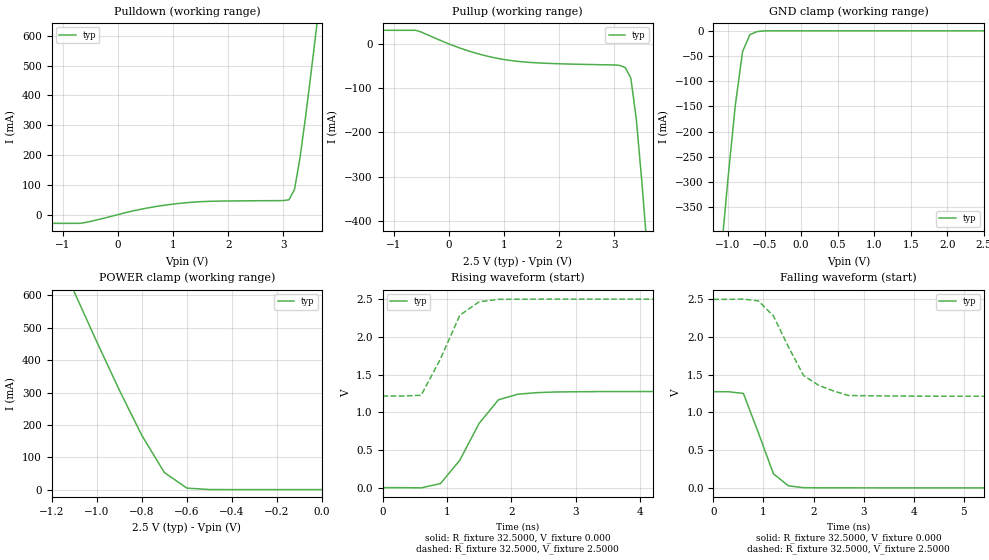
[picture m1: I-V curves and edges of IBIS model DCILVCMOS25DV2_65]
| / 7\'7
| \ \   Xilinx Inc.
| / /
| \_\/.\   IBIS Model for Virtex-II
[IBIS ver]   2.1
[File name]   dci2565d.ibs
[File Rev]   1.1
[Date]   Aug. 1, 2001
[Source]   Hspice simulations (08-01: TT, SS, FF)
[Notes]   Xilinx IBIS model for LVDCI 2.5V 32.5 ohms (65/2) driver
[Disclaimer] The data in this model is derived from SPICE simulations using
   modeling information extracted from the target process. While
   a great deal of care has been taken to provide information
   that is accurate, this model is considered preliminary as it
   has not been verified by actual silicon measurement. Treat the
   data in this model as preliminary until actual silicon
   verification is performed.
[Copyright]   Copyright 2001, Xilinx Inc., All rights reserved
|   Component Virtex_II
[Component]   Virtex_II
[Manufacturer]   Xilinx Inc.
[Package]
| variable   typ   min   max
R_pkg   0.1000   NA   NA
L_pkg   0.8000nH   NA   NA
C_pkg   0.5000pF   NA   NA
[Pin]  signal_name   model_name   R_pin   L_pin   C_pin
io   DCILVCMOS25DV2_65   DCILVCMOS25DV2_65
| ins  insig   inp
| ens  ensig   inp
PGND   GND   GND
VCCO   VCCO   POWER
| Models and submodels in the file (1): DCILVCMOS25DV2_65 (I/O)
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|   Model DCILVCMOS25DV2_65
[Model]   DCILVCMOS25DV2_65
Model_type   I/O
Polarity   Non-Inverting
Enable   Active-Low
Vinh = 1.7V
Vinl = 0.7V
Vmeas =   1.2000V
Cref =  35.0000pF
Rref =   1.0000M
Vref =  0.000V
C_comp   7.0000pF   NA   NA
[Temperature Range]   25.0000   NA   NA
[Voltage Range]   2.5000V   NA   NA
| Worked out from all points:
|   slope of the pulldown table from 0 to 0.375 V, typ, clamps not added: 22.9 ohm
|   slope of the pullup table from 0 to 0.375 V, typ, clamps not added: 22.5 ohm
|   GND clamp passes 1 mA (typ) near -0.57 V on its own axis
|   POWER clamp passes 1 mA (typ) near -0.52 V on its own axis
|   rising waveform, R_fixture 32.5000, V_fixture 0.000: 20-80 % time 566ps typ, NA min, NA max; typ from 0 V to 1.27 V
|   rising waveform, R_fixture 32.5000, V_fixture 2.5000: 20-80 % time 424ps typ, NA min, NA max; typ from 1.22 V to 2.5 V
|   falling waveform, R_fixture 32.5000, V_fixture 0.000: 20-80 % time 429ps typ, NA min, NA max; typ from 1.27 V to 0 V
|   falling waveform, R_fixture 32.5000, V_fixture 2.5000: 20-80 % time 617ps typ, NA min, NA max; typ from 2.5 V to 1.22 V
[Pulldown]
| voltage   I(typ)   I(min)   I(max)
-2.5V     -29.43mA   NA         NA
-700mV    -29.43mA   NA         NA
400mV     17.34mA    NA         NA
1.1V      37.38mA    NA         NA
1.6V      44.23mA    NA         NA
3.1V      49.76mA    NA         NA
3.2V      84.49mA    NA         NA
3.3V      190.6mA    NA         NA
3.4V      327.7mA    NA         NA
3.5V      475.6mA    NA         NA
3.6V      628.9mA    NA         NA
5V        2.891A     NA         NA
[Pullup]
| voltage   I(typ)   I(min)   I(max)
-2.5V     30.51mA    NA         NA
-600mV    30.51mA    NA         NA
300mV     -13.68mA   NA         NA
900mV     -33.24mA   NA         NA
1.6V      -42.95mA   NA         NA
3V        -47.71mA   NA         NA
3.2V      -53.72mA   NA         NA
3.3V      -77.44mA   NA         NA
3.4V      -171.4mA   NA         NA
3.5V      -312.3mA   NA         NA
3.6V      -469.3mA   NA         NA
5V        -2.896A    NA         NA
[GND_clamp]
| voltage   I(typ)   I(min)   I(max)
-2.5V     -2.881A    NA         NA
-1.1V     -452.1mA   NA         NA
-1V       -293.4mA   NA         NA
-900mV    -148.1mA   NA         NA
-800mV    -41.04mA   NA         NA
-700mV    -7.632mA   NA         NA
-600mV    -1.432mA   NA         NA
-500mV    -131.2uA   NA         NA
2.5V      397.5nA    NA         NA
[POWER_clamp]
| voltage   I(typ)   I(min)   I(max)
-2.5V     2.874A     NA         NA
-1.1V     610.9mA    NA         NA
-1V       456.9mA    NA         NA
-900mV    307.7mA    NA         NA
-800mV    167.5mA    NA         NA
-700mV    52.78mA    NA         NA
-600mV    4.607mA    NA         NA
-500mV    279.3uA    NA         NA
0V        397.5nA    NA         NA
[Ramp]
| variable   typ   min   max
dV/dt_r   0.7650/0.5000n   NA   NA
dV/dt_f   0.7710/0.6731n   NA   NA
R_load = 32.5000
[Rising Waveform]
R_fixture = 32.5000
V_fixture = 0.000
| time   V(typ)   V(min)   V(max)
0s        6.382uV    NA         NA
600ps     -2.675mV   NA         NA
900ps     54.08mV    NA         NA
1.2ns     363.1mV    NA         NA
1.5ns     852.3mV    NA         NA
1.8ns     1.165V     NA         NA
2.1ns     1.239V     NA         NA
2.7ns     1.269V     NA         NA
3.6ns     1.275V     NA         NA
15ns      1.275V     NA         NA
[Rising Waveform]
R_fixture = 32.5000
V_fixture = 2.5000
V_fixture_min = 2.3000
V_fixture_max = 2.7000
| time   V(typ)   V(min)   V(max)
0s        1.215V     NA         NA
300ps     1.215V     NA         NA
600ps     1.225V     NA         NA
900ps     1.708V     NA         NA
1.2ns     2.286V     NA         NA
1.5ns     2.464V     NA         NA
1.8ns     2.498V     NA         NA
15ns      2.5V       NA         NA
[Falling Waveform]
R_fixture = 32.5000
V_fixture = 0.000
| time   V(typ)   V(min)   V(max)
0s        1.275V     NA         NA
300ps     1.275V     NA         NA
600ps     1.252V     NA         NA
900ps     728.6mV    NA         NA
1.2ns     186.6mV    NA         NA
1.5ns     26.61mV    NA         NA
1.8ns     2.612mV    NA         NA
2.1ns     826.2uV    NA         NA
15ns      5.956uV    NA         NA
[Falling Waveform]
R_fixture = 32.5000
V_fixture = 2.5000
V_fixture_min = 2.3000
V_fixture_max = 2.7000
| time   V(typ)   V(min)   V(max)
0s        2.5V       NA         NA
600ps     2.503V     NA         NA
900ps     2.479V     NA         NA
1.2ns     2.28V      NA         NA
1.5ns     1.869V     NA         NA
1.8ns     1.491V     NA         NA
2.1ns     1.361V     NA         NA
2.7ns     1.224V     NA         NA
4.5ns     1.215V     NA         NA
15ns      1.215V     NA         NA
